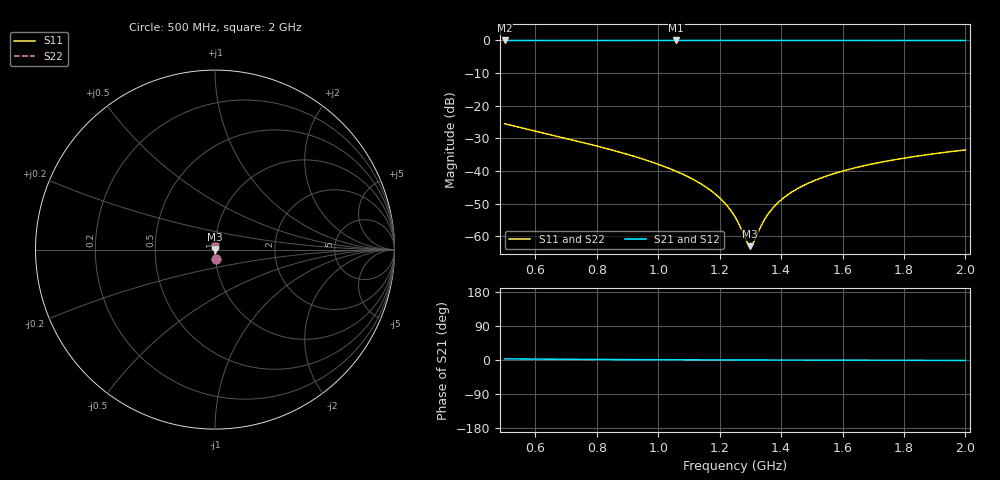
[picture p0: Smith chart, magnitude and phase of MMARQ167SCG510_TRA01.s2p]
! MMARQ167SCG510_TRA01  S-PARAMETER MODEL  ( General Type )
! Model Generated by TAIYO YUDEN Corporation (http://www.ty-top.com)
! Version 1.0
! TAIYO YUDEN Control No. 160201
! Copyright(c) 2016 TAIYO YUDEN CO.,LTD. All Rights Reserved.
! Product Description (link to TY-COMPAS)
! https://ds.yuden.co.jp/TYCOMPAS/or/detail?pn=MMARQ167SCG510JTRA01&u=M
! Products Name : Multilayer Ceramic Capacitors
! Characteristics :
!  Capacitance : 51 pF , Rated Voltage : 250V , TCC : CG / C0G
!  Case Size : 1.6 x 0.8 / 0.063 x 0.031 [mm/inch] , Thickness : 0.7 / 0.028 [mm/inch]
!  (Conditions: Temperature = 25 degC , DC Bias Current/Voltage = 0A / 0V)
! External Node Assignments :
!  1  o---| |---o  2
! GND o---------o GND
! Frequency Range : 500MHz  -  2000MHz  [ 401 STEP ]
# MHz S RI R 50
! Freq[MHz].  S11 Real  S11 Imag  S21 Real  S21 Imag  S12 Real  S12 Imag  S22 Real  S22 Imag
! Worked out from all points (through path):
!   401 points, 500 MHz to 2 GHz, reference 50 ohm
!   highest |S21| = -0.01 dB at 1.059 GHz (marker M1); lowest = 0.0 dB at 500 MHz (marker M2)
!   lowest |S11| = -63.0 dB at 1.299 GHz (marker M3), VSWR 1.00, Z = 50.1 - j0.00512 ohm
!   |S11| at or under -10 dB: start of sweep to end of sweep
!   |S22| runs from -63.0 to -25.5 dB; largest |S21 - S12| = 0
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500  0.00322 -0.0531  0.9968 0.0531  0.9968 0.0531  0.00322 -0.0531
751.25  0.00123 -0.0276  0.9988 0.0276  0.9988 0.0276  0.00123 -0.0276
893.75  0.000857 -0.0184  0.9991 0.0184  0.9991 0.0184  0.000857 -0.0184
1002.5  0.000724 -0.0126  0.9993 0.0126  0.9993 0.0126  0.000724 -0.0126
1058.75  0.000689 -0.0099  0.9993 0.0099  0.9993 0.0099  0.000689 -0.0099
1122.5  0.000671 -0.00705  0.9993 0.00705  0.9993 0.00705  0.000671 -0.00705
1175  0.00067 -0.00485  0.9993 0.00485  0.9993 0.00485  0.00067 -0.00485
1216.25  0.000677 -0.00319  0.9993 0.00319  0.9993 0.00319  0.000677 -0.00319
1250  0.000687 -0.00188  0.9993 0.00188  0.9993 0.00188  0.000687 -0.00188
1265  0.000693 -0.00131  0.9993 0.00131  0.9993 0.00131  0.000693 -0.00131
1287.5  0.000703 -0.000467  0.9993 0.000467  0.9993 0.000467  0.000703 -0.000467
1298.75  0.000708 -5.11e-05  0.9993 5.11e-05  0.9993 5.11e-05  0.000708 -5.11e-05
1302.5  0.00071 8.66e-05  0.9993 -8.66e-05  0.9993 -8.66e-05  0.00071 8.66e-05
1310  0.000714 0.000361  0.9993 -0.000361  0.9993 -0.000361  0.000714 0.000361
1336.25  0.00073 0.00131  0.9993 -0.00131  0.9993 -0.00131  0.00073 0.00131
1351.25  0.000739 0.00184  0.9993 -0.00184  0.9993 -0.00184  0.000739 0.00184
1381.25  0.00076 0.00289  0.9992 -0.00289  0.9992 -0.00289  0.00076 0.00289
1433.75  0.000801 0.00467  0.9992 -0.00467  0.9992 -0.00467  0.000801 0.00467
1501.25  0.000863 0.00688  0.9991 -0.00688  0.9991 -0.00688  0.000863 0.00688
1610  0.000981 0.0103  0.999 -0.0103  0.999 -0.0103  0.000981 0.0103
1752.5  0.00116 0.0144  0.9988 -0.0144  0.9988 -0.0144  0.00116 0.0144
2000  0.00154 0.0211  0.9985 -0.0211  0.9985 -0.0211  0.00154 0.0211
